|   IBIS Model for AM1802ZCE
[IBIS Ver]   3.2
[Comment Char]  |_char
[File Name]   AM1802_zce.ibs
[File Rev]   1.0
[Date]   March 8, 2013
[Source]   From Optimal Corporation's PakSi-E result.
[Notes]   Created from Freon_16x16_OSV_12172008_H_1.mcm
|   (1) AM1802 ZCE contains dual rail I/O buffers that
|   are capable of running are two different core
|   voltages depedent on the schematic hookup
|   (a) 1.8V
|   (b) 3.3V
|   (2) Specific Model Sections/Name Decoders are determined
|   based upon the value that is supplied to the
|   particular I/O buffer as well as any pull up/down
|   resistors that are selected. Refer to the Model Selecter
|   Definitions for details regarding model selection at
|   1.8V rail or the 3.3V rail.
[Disclaimer]
|   Please be aware that in the absence of a written agreement
|   Texas Instruments (TI) assumes no liability for:
|   (1) The accuracy of the IBIS models provided to your company
|   (2) The proper functioning of these Models in your design
|   or for any resulting applications;or
|   (3) Infringement of patents,copyrights, or intellectual
|   property rights resulting from your use of these models.
|   TI provides IBIS Models as a service to our customers and
|   therefore reserves the right to limit distribution of the
|   Models.
[Copyright] Copyright 2011, Texas Instruments Incorporated. All Rights Reserved
[Component]   AM1802ZCE
[Manufacturer]   Texas Instruments
[Package]
| variable   typ   min   max
R_pkg   4.15668e-001  2.28452e-002  6.49659e-001
L_pkg   3.30265e-009  8.15850e-011  6.01630e-009
C_pkg   7.30249e-013  5.00661e-013  1.13139e-012
| Note - some signal_names were truncated to meet the 80 character
|  per line limit of IBIS spec v3.2
[Pin] signal_name  model_name R_pin   L_pin   C_pin
A1   ACLKR_GP015  BC1833DV40CTPBFZ 5.91871e-001 5.89640e-009 8.85863e-013
B1   ACLKX_GP014  BC1833DV40CTPBFZ 4.86257e-001 5.42480e-009 8.43455e-013
C2   AFSR0_GP013  BC1833DV40CTPBFZ 4.95087e-001 4.50480e-009 8.94184e-013
B2   AFSX0_GP012  BC1833DV40CTPBFZ 5.24155e-001 4.89370e-009 9.02440e-013
A2   AHCLKR   BC1833DV40CTPBFZ 5.57738e-001 5.17010e-009 9.36823e-013
A3   AHCLKX   BC1833DV40CTPBFZ 6.49659e-001 6.01630e-009 1.04360e-012
D5   AMUTE   BC1833DV40CTPBFZ 5.05628e-001 3.54900e-009 1.13139e-012
F4   AMUTEIN   BC1833DV40CTPBFZ 2.70359e-001 2.09390e-009 8.60715e-013
F3   AXR00   BC1833DV40CTPBFZ 5.87268e-001 5.04320e-009 8.85130e-013
E1   AXR01   BC1833DV40CTPBFZ 5.06257e-001 4.56730e-009 7.02096e-013
D4   AXR010   BC1833DV40CTPBFZ 4.50538e-001 2.95250e-009 9.90146e-013
C5   AXR011   BC1833DV40CTPBFZ 2.58059e-001 2.51010e-009 8.40608e-013
C4   AXR012   BC1833DV40CTPBFZ 4.53251e-001 3.15490e-009 8.42999e-013
B3   AXR013   BC1833DV40CTPBFZ 4.94703e-001 4.00220e-009 7.40491e-013
B4   AXR014   BC1833DV40CTPBFZ 6.26064e-001 5.27040e-009 8.70708e-013
A4   AXR015   BC1833DV40CTPBFZ 5.69193e-001 4.65980e-009 7.60530e-013
E2   AXR02   BC1833DV40CTPBFZ 4.58046e-001 4.05840e-009 7.62216e-013
E3   AXR03   BC1833DV40CTPBFZ 6.03822e-001 5.34400e-009 9.04861e-013
D1   AXR04   BC1833DV40CTPBFZ 5.22228e-001 4.82720e-009 7.59112e-013
D3   AXR05   BC1833DV40CTPBFZ 6.17668e-001 5.68500e-009 9.46537e-013
C1   AXR06   BC1833DV40CTPBFZ 5.46060e-001 5.18360e-009 7.72304e-013
D2   AXR07   BC1833DV40CTPBFZ 4.69058e-001 4.07530e-009 8.16364e-013
E4   AXR08   BC1833DV40CTPBFZ 4.33873e-001 2.99390e-009 9.65579e-013
C3   AXR09   BC1833DV40CTPBFZ 4.41997e-001 3.42670e-009 8.54225e-013
C14  EMAA0_GP50   BC1833DV40CTPBFZ 2.98382e-001 2.12110e-009 6.59617e-013
D15  EMAA1_GP51   BC1833DV40CTPBFZ 5.42787e-001 4.38610e-009 7.97764e-013
C12  EMAA10_GP510 BC1833DV40CTPBFZ 2.66169e-001 1.88560e-009 6.21067e-013
B12  EMAA11_GP511 BC1833DV40CTPBFZ 2.63919e-001 2.25010e-009 6.03279e-013
D13  EMAA12_GP512 BC1833DV40CTPBFZ 4.96551e-001 4.38480e-009 8.15026e-013
D11  EMAA13_GP513 BC1833DV40CTPBFZ 4.28105e-001 2.84370e-009 7.34402e-013
A12  EMAA14_GP514 BC1833DV40CTPBFZ 3.52992e-001 3.00810e-009 5.84119e-013
C11  EMAA15_GP515 BC1833DV40CTPBFZ 2.52056e-001 1.79990e-009 6.53107e-013
E12  EMAA16_GP40  BC1833DV40CTPBFZ 5.25507e-001 4.62630e-009 8.90034e-013
B11  EMAA17_GP41  BC1833DV40CTPBFZ 3.48210e-001 2.51590e-009 6.11958e-013
E11  EMAA18_GP42  BC1833DV40CTPBFZ 4.54964e-001 3.32960e-009 8.69791e-013
C10  EMAA19_GP43  BC1833DV40CTPBFZ 3.76906e-001 2.39340e-009 7.09774e-013
B14  EMAA2_GP52   BC1833DV40CTPBFZ 3.90592e-001 2.72300e-009 6.24758e-013
A11  EMAA20_GP44  BC1833DV40CTPBFZ 3.45761e-001 2.96740e-009 6.10012e-013
B10  EMAA21_GP45  BC1833DV40CTPBFZ 2.46960e-001 2.00900e-009 5.42935e-013
A10  EMAA22_GP46  BC1833DV40CTPBFZ 3.33152e-001 2.60470e-009 5.37496e-013
E9   EMAA23_GP47  BC1833DV40CTPBFZ 3.19065e-001 2.29880e-009 7.32743e-013
D14  EMAA3_GP53   BC1833DV40CTPBFZ 4.79376e-001 3.69480e-009 7.71487e-013
A14  EMAA4_GP54   BC1833DV40CTPBFZ 3.97984e-001 3.13500e-009 5.42094e-013
C13  EMAA5_GP55   BC1833DV40CTPBFZ 4.22523e-001 2.74470e-009 6.79880e-013
E13  EMAA6_GP56   BC1833DV40CTPBFZ 3.48995e-001 2.90190e-009 8.13518e-013
B13  EMAA7_GP57   BC1833DV40CTPBFZ 3.66929e-001 2.60810e-009 6.24751e-013
A13  EMAA8_GP58   BC1833DV40CTPBFZ 3.72708e-001 3.04190e-009 5.38465e-013
D12  EMAA9_GP59   BC1833DV40CTPBFZ 3.33588e-001 2.40090e-009 7.00953e-013
C15  EMABA0_GP28  BC1833DV40CTPBFZ 3.18300e-001 2.38740e-009 7.10753e-013
A15  EMABA1_GP29  BC1833DV40CTPBFZ 4.17096e-001 3.30950e-009 5.86538e-013
A9   EMACASn_GP24 BC1833DV40CTPBFZ 3.54881e-001 2.82330e-009 5.65088e-013
B7   EMACLK_GP27  BC1833DV40CTPBFZ 3.56531e-001 2.34950e-009 5.60045e-013
A18  EMACS0n_GP20 BC1833DV40CTPBFZ 3.97081e-001 3.74280e-009 7.21563e-013
B17  EMACS2n_GP315 BC1833DV40CTPBFZ 5.80198e-001 5.09880e-009 8.43227e-013
A17  EMACS3n_GP314 BC1833DV40CTPBFZ 3.78016e-001 3.46170e-009 7.23538e-013
F9   EMACS4n_GP313 BC1833DV40CTPBFZ 5.19550e-001 3.90300e-009 9.18755e-013
B16  EMACS5n_GP212 BC1833DV40CTPBFZ 5.51095e-001 4.76040e-009 7.96121e-013
C9   EMAD0_GP48   BC1833DV40CTPBFZ 2.44304e-001 1.64890e-009 6.18740e-013
A8   EMAD1_GP49   BC1833DV40CTPBFZ 3.32250e-001 2.52330e-009 5.06368e-013
A7   EMAD10_GP32  BC1833DV40CTPBFZ 3.48770e-001 2.64970e-009 5.08237e-013
D6   EMAD11_GP33  BC1833DV40CTPBFZ 2.37569e-001 1.57190e-009 7.49192e-013
A6   EMAD12_GP34  BC1833DV40CTPBFZ 5.66268e-001 4.40960e-009 8.45128e-013
B6   EMAD13_GP35  BC1833DV40CTPBFZ 5.13874e-001 3.70700e-009 7.90354e-013
C7   EMAD14_GP36  BC1833DV40CTPBFZ 5.91744e-001 4.61700e-009 1.00047e-012
E6   EMAD15_GP37  BC1833DV40CTPBFZ 1.98115e-001 1.36540e-009 7.81085e-013
B8   EMAD2_GP410  BC1833DV40CTPBFZ 3.46727e-001 2.30150e-009 5.60570e-013
E8   EMAD3_GP411  BC1833DV40CTPBFZ 4.91407e-001 3.76040e-009 8.64890e-013
B5   EMAD4_GP412  BC1833DV40CTPBFZ 4.54268e-001 3.17380e-009 6.52985e-013
E7   EMAD5_GP413  BC1833DV40CTPBFZ 2.62992e-001 2.12650e-009 1.09788e-012
C6   EMAD6_GP414  BC1833DV40CTPBFZ 5.38100e-001 3.95790e-009 8.47380e-013
D7   EMAD7_GP415  BC1833DV40CTPBFZ 5.81194e-001 4.67290e-009 1.06233e-012
E10  EMAD8_GP30   BC1833DV40CTPBFZ 3.75790e-001 3.17900e-009 8.92133e-013
D9   EMAD9_GP31   BC1833DV40CTPBFZ 4.95004e-001 3.95170e-009 7.99211e-013
B15  EMAOEn_GP310 BC1833DV40CTPBFZ 2.95177e-001 2.25360e-009 5.63438e-013
A16  EMARASn_GP25 BC1833DV40CTPBFZ 4.31087e-001 3.59950e-009 5.83703e-013
D10  EMARNW_GP39  BC1833DV40CTPBFZ 4.67072e-001 3.80790e-009 7.79641e-013
D8   EMASDCKE_GP26 BC1833DV40CTPBFZ 4.66445e-001 3.42630e-009 7.54319e-013
B18  EMAWAIT0_GP38 BC1833DV40CTPBFZ 4.09634e-001 3.45430e-009 7.14985e-013
B19  EMAWAIT1_GP21 BC1833DV40CTPBFZ 4.41357e-001 4.08480e-009 8.09083e-013
B9   EMAWEn_GP311 BC1833DV40CTPBFZ 3.54014e-001 2.53790e-009 5.62877e-013
C8   EMAWEDQM0n_GP23 BC1833DV40CTPBFZ 3.74193e-001 2.37840e-009 6.26113e-013
A5   EMAWEDQM1n_GP22 BC1833DV40CTPBFZ 5.13242e-001 3.94230e-009 6.49289e-013
U7   DDRA0   BSSTL18TCSCGPBFZ 4.14960e-001 2.73750e-009 6.79471e-013
T7   DDRA1   BSSTL18TCSCGPBFZ 4.61192e-001 3.10260e-009 7.39296e-013
W6   DDRA2   BSSTL18TCSCGPBFZ 3.98765e-001 3.02010e-009 5.57871e-013
V6   DDRA3   BSSTL18TCSCGPBFZ 2.72035e-001 2.08680e-009 5.20945e-013
U5   DDRA4   BSSTL18TCSCGPBFZ 4.39992e-001 3.22490e-009 6.44839e-013
V5   DDRA5   BSSTL18TCSCGPBFZ 4.35683e-001 3.07040e-009 5.81074e-013
W5   DDRA6   BSSTL18TCSCGPBFZ 4.21472e-001 3.27020e-009 5.67079e-013
U6   DDRA7   BSSTL18TCSCGPBFZ 2.85462e-001 1.89380e-009 6.46976e-013
U4   DDRA8   BSSTL18TCSCGPBFZ 4.88010e-001 3.63800e-009 7.05605e-013
T6   DDRA9   BSSTL18TCSCGPBFZ 1.92149e-001 1.42270e-009 6.24918e-013
W4   DDRA10   BSSTL18TCSCGPBFZ 4.35328e-001 3.47630e-009 5.60660e-013
T4   DDRA11   BSSTL18TCSCGPBFZ 5.10405e-001 3.72920e-009 8.12116e-013
V4   DDRA12   BSSTL18TCSCGPBFZ 4.38115e-001 3.08480e-009 5.82197e-013
T5   DDRA13   BSSTL18TCSCGPBFZ 2.15693e-001 1.70520e-009 7.47184e-013
V8   DDRBA0   BSSTL18TCSCGPBFZ 4.80522e-001 3.52320e-009 6.92654e-013
T9   DDRBA1   BSSTL18TCSCGPBFZ 2.20318e-001 1.65540e-009 6.83534e-013
U8   DDRBA2   BSSTL18TCSCGPBFZ 4.04014e-001 2.49850e-009 6.68341e-013
U9   DDRCASn   BSSTL18TCSCGPBFZ 3.88058e-001 2.44280e-009 6.26800e-013
V7   DDRCKE   BSSTL18TCSCGPBFZ 2.57587e-001 2.00620e-009 5.46471e-013
W7   DDRCLKN   BSSTL18TCSCGPBFZ 3.64269e-001 2.70550e-009 5.00661e-013
W8   DDRCLKP   BSSTL18TCSCGPBFZ 3.53476e-001 2.69690e-009 5.06199e-013
V9   DDRCSn   BSSTL18TCSCGPBFZ 3.47483e-001 2.33680e-009 5.61910e-013
U15  DDRD0   BSSTL18TCSCGPBFZ 5.03067e-001 4.08480e-009 6.88721e-013
U14  DDRD1   BSSTL18TCSCGPBFZ 4.44055e-001 3.34930e-009 6.99179e-013
V14  DDRD2   BSSTL18TCSCGPBFZ 4.43485e-001 3.67420e-009 6.49287e-013
U13  DDRD3   BSSTL18TCSCGPBFZ 4.23858e-001 3.01220e-009 6.42646e-013
V13  DDRD4   BSSTL18TCSCGPBFZ 2.95715e-001 2.54430e-009 6.14396e-013
V12  DDRD5   BSSTL18TCSCGPBFZ 3.88855e-001 2.74710e-009 5.41742e-013
W12  DDRD6   BSSTL18TCSCGPBFZ 3.67182e-001 2.92840e-009 5.28344e-013
W11  DDRD7   BSSTL18TCSCGPBFZ 2.56622e-001 2.82530e-009 6.12911e-013
T13  DDRD8   BSSTL18TCSCGPBFZ 4.76155e-001 3.51100e-009 8.24674e-013
T11  DDRD9   BSSTL18TCSCGPBFZ 4.46810e-001 3.14220e-009 7.61080e-013
T10  DDRD10   BSSTL18TCSCGPBFZ 3.12174e-001 2.45150e-009 6.81267e-013
T12  DDRD11   BSSTL18TCSCGPBFZ 4.66794e-001 3.38780e-009 8.50234e-013
U10  DDRD12   BSSTL18TCSCGPBFZ 3.86652e-001 2.58760e-009 6.64029e-013
V10  DDRD13   BSSTL18TCSCGPBFZ 3.78944e-001 2.51470e-009 6.06810e-013
U11  DDRD14   BSSTL18TCSCGPBFZ 4.74936e-001 3.29650e-009 8.05328e-013
W10  DDRD15   BSSTL18TCSCGPBFZ 3.79744e-001 3.73260e-009 6.60169e-013
W13  DDRDQM0n   BSSTL18TCSCGPBFZ 3.94835e-001 3.04360e-009 5.62703e-013
R10  DDRDQM1n   BSSTL18TCSCGPBFZ 4.61673e-001 3.54330e-009 8.26589e-013
W9   DDRRASn   BSSTL18TCSCGPBFZ 3.50051e-001 2.72800e-009 5.47279e-013
R11  DDRDQGATE0   BSSTL18TCSCGPBFZ 4.90814e-001 3.50590e-009 8.76801e-013
R12  DDRDQGATE1   BSSTL18TCSCGPBFZ 5.15291e-001 3.70680e-009 9.84983e-013
T8   DDRWEn   BSSTL18TCSCGPBFZ 4.42497e-001 2.97360e-009 6.63102e-013
T14  DDRDQS0   BSSTL18TCSCGPBFZ 4.80092e-001 3.48030e-009 7.80760e-013
V11  DDRDQS1   BSSTL18TCSCGPBFZ 4.22650e-001 3.29520e-009 6.81403e-013
J16  EMU0   BC1833DV40CTPBFZ 2.54325e-001 1.81840e-009 7.85509e-013
K16  EMU1   BC1833DV40CTPBFZ 4.29846e-001 3.27960e-009 8.14633e-013
K4   GP61   BC1833DV40CTPBFZ 3.63614e-001 2.49020e-009 8.31825e-013
J3   GP62   BC1833DV40CTPBFZ 2.73739e-001 2.52640e-009 7.69287e-013
K3   GP63   BC1833DV40CTPBFZ 3.69454e-001 2.75510e-009 7.14832e-013
H3   GP64   BC1833DV40CTPBFZ 5.80089e-001 5.21570e-009 8.91399e-013
F2   GP810   BC1833DV40CTPBFZ 4.49068e-001 3.95750e-009 7.41073e-013
F1   GP811   BC1833DV40CTPBFZ 4.97064e-001 4.59930e-009 7.63107e-013
G3   GP812   BC1833DV40CTPBFZ 4.22225e-001 3.12280e-009 9.06650e-013
J4   GP813   BC1833DV40CTPBFZ 4.18358e-001 2.77620e-009 8.64397e-013
G2   GP814   BC1833DV40CTPBFZ 4.46474e-001 3.75040e-009 7.54261e-013
G1   GP815   BC1833DV40CTPBFZ 4.80067e-001 4.12220e-009 6.81038e-013
G4   GP88   BC1833DV40CTPBFZ 3.97460e-001 2.83360e-009 8.04305e-013
H4   GP89   BC1833DV40CTPBFZ 4.23690e-001 2.97660e-009 8.22397e-013
R5   GP60   BC1833DV40CTPBFZ 2.45883e-001 2.09100e-009 8.01025e-013
W1   GP78   BC1833DV40CTPBFZ 4.78964e-001 4.27560e-009 6.54315e-013
W2   GP79   BC1833DV40CTPBFZ 4.54813e-001 3.82070e-009 6.79498e-013
T2   GP72   BC1833DV40CTPBFZ 4.36957e-001 3.45270e-009 5.91877e-013
T3   GP73   BC1833DV40CTPBFZ 4.16931e-001 3.05630e-009 6.29650e-013
R1   GP74   BC1833DV40CTPBFZ 4.54506e-001 3.65190e-009 6.34173e-013
R2   GP75   BC1833DV40CTPBFZ 4.20647e-001 3.27220e-009 7.29881e-013
R3   GP76   BC1833DV40CTPBFZ 3.26617e-001 2.78190e-009 6.90042e-013
P4   GP77   BC1833DV40CTPBFZ 4.14093e-001 2.81750e-009 7.64469e-013
W3   GP710   BC1833DV40CTPBFZ 2.28452e-002 1.01420e-010 5.62555e-013
V1   GP711   BC1833DV40CTPBFZ 4.77687e-001 4.00580e-009 6.74578e-013
V2   GP712   BC1833DV40CTPBFZ 4.48597e-001 3.75400e-009 6.51164e-013
V3   GP713   BC1833DV40CTPBFZ 4.36018e-001 3.43390e-009 7.00041e-013
U1   GP714   BC1833DV40CTPBFZ 4.80254e-001 3.78490e-009 6.52073e-013
U2   GP715   BC1833DV40CTPBFZ 4.40999e-001 3.40200e-009 6.15258e-013
U3   GP70   BC1833DV40CTPBFZ 4.34081e-001 3.33150e-009 6.89105e-013
T1   GP71   BC1833DV40CTPBFZ 4.87422e-001 3.88830e-009 5.92797e-013
J17  NMIn   IC1833DVTPBFZP18LL 3.65961e-001 2.64340e-009 6.81345e-013
K14  RESETn   IHHV1833DVTP18 3.13948e-001 1.92720e-009 9.39463e-013
K17  GP80   BC1833DV40CTPBFZ 4.98560e-001 4.09850e-009 7.97021e-013
D19  EPWM0A   BC1833DV40CTPBFZ 5.47450e-001 4.73470e-009 7.69394e-013
C17  EPWM0B   BC1833DV40CTPBFZ 2.77268e-001 2.63370e-009 7.30178e-013
D17  GP16   BC1833DV40CTPBFZ 4.00877e-001 2.84850e-009 6.63256e-013
E16  GP17   BC1833DV40CTPBFZ 1.85753e-001 1.58290e-009 7.38386e-013
D16  GP81   BC1833DV40CTPBFZ 2.94303e-001 2.04320e-009 6.93329e-013
E17  GP82   BC1833DV40CTPBFZ 4.47987e-001 3.34480e-009 7.84496e-013
D18  GP83   BC1833DV40CTPBFZ 4.37452e-001 3.53960e-009 6.89681e-013
C19  GP84   BC1833DV40CTPBFZ 4.72581e-001 3.82440e-009 6.65189e-013
C18  GP85   BC1833DV40CTPBFZ 4.70155e-001 3.77380e-009 6.89104e-013
C16  GP86   BC1833DV40CTPBFZ 2.76089e-001 2.46530e-009 7.57539e-013
G19  SPI1CLK_GP213 BC1833DV40CTPBFZ 4.69262e-001 4.17240e-009 7.11445e-013
H16  SPI1ENAn_GP212 BC1833DV40CTPBFZ 2.65537e-001 2.13550e-009 7.16472e-013
E19  SPI1SCS0n   BC1833DV40CTPBFZ 4.90496e-001 4.15100e-009 7.37763e-013
F18  SPI1SCS1n   BC1833DV40CTPBFZ 4.59876e-001 3.78990e-009 7.28257e-013
F19  SPI1SCS2n   BC1833DV40CTPBFZ 4.93949e-001 4.19790e-009 7.59046e-013
E18  SPI1SCS3n   BC1833DV40CTPBFZ 3.81442e-001 3.01750e-009 6.17218e-013
F16  SPI1SCS4n   BC1833DV40CTPBFZ 3.91821e-001 2.59160e-009 7.64737e-013
F17  SPI1SCS5n   BC1833DV40CTPBFZ 3.81978e-001 2.67900e-009 6.57715e-013
G18  SPI1SCS6n   BC1833DV40CTPBFZ 4.07238e-001 3.79210e-009 7.95139e-013
G16  SPI1SCS7n   BC1833DV40CTPBFZ 2.69265e-001 1.90170e-009 7.00785e-013
G17  SPI1SIMO_GP210 BC1833DV40CTPBFZ 3.72117e-001 2.60560e-009 6.80138e-013
H17  SPI1SOMI_GP211 BC1833DV40CTPBFZ 4.56903e-001 3.42860e-009 7.28034e-013
J15  TCK   IC1833DVTPBFZP18LL 2.57521e-001 1.72010e-009 7.51806e-013
M16  TDI   IC1833DVTPBFZP18LL 5.58912e-001 5.27220e-009 1.06666e-012
J18  TDO   BC1833DV40CTPBFZ 3.51274e-001 2.87560e-009 6.76444e-013
L16  TMS   IC1833DVTPBFZP18LL 3.99407e-001 2.92060e-009 8.37004e-013
L17  TRSTn   IC1833DVTPBFZP18LL 3.86978e-001 3.09900e-009 7.62159e-013
T17  UHPIHASn   BC1833DV40CTPBFZ 3.86492e-001 2.71460e-009 7.41946e-013
U17  UHPIHCNTL0   BC1833DV40CTPBFZ 2.42945e-002 8.15850e-011 8.17122e-013
W15  UHPIHCNTL1   BC1833DV40CTPBFZ 4.27573e-001 3.54430e-009 5.42549e-013
W14  UHPIHCSn   BC1833DV40CTPBFZ 3.48379e-001 3.02510e-009 5.61183e-013
P17  UHPIHD0   BC1833DV40CTPBFZ 5.04430e-001 4.02180e-009 9.65050e-013
R15  UHPIHD1   BC1833DV40CTPBFZ 4.61967e-001 3.22070e-009 9.22461e-013
W17  UHPIHD10   BC1833DV40CTPBFZ 5.06372e-001 4.43790e-009 6.29295e-013
V17  UHPIHD11   BC1833DV40CTPBFZ 5.14141e-001 4.40180e-009 6.46147e-013
W16  UHPIHD12   BC1833DV40CTPBFZ 4.47674e-001 3.61480e-009 5.80945e-013
R14  UHPIHD13   BC1833DV40CTPBFZ 2.29936e-001 1.93580e-009 9.83864e-013
V16  UHPIHD14   BC1833DV40CTPBFZ 4.88188e-001 3.91970e-009 6.17589e-013
U18  UHPIHD15   BC1833DV40CTPBFZ 5.62311e-001 4.83050e-009 8.64648e-013
R19  UHPIHD2   BC1833DV40CTPBFZ 5.16823e-001 4.57930e-009 7.51770e-013
R18  UHPIHD3   BC1833DV40CTPBFZ 5.00110e-001 4.15440e-009 7.75793e-013
T16  UHPIHD4   BC1833DV40CTPBFZ 2.66853e-001 2.25470e-009 8.85923e-013
U19  UHPIHD5   BC1833DV40CTPBFZ 5.90890e-001 5.06810e-009 8.95998e-013
V19  UHPIHD6   BC1833DV40CTPBFZ 5.79160e-001 4.93500e-009 7.59523e-013
V18  UHPIHD7   BC1833DV40CTPBFZ 5.37053e-001 4.49240e-009 8.46758e-013
W19  UHPIHD8   BC1833DV40CTPBFZ 5.52593e-001 5.15440e-009 7.41144e-013
W18  UHPIHD9   BC1833DV40CTPBFZ 5.25636e-001 4.65020e-009 7.16361e-013
V15  UHPIHDS1n   BC1833DV40CTPBFZ 3.19300e-001 2.53200e-009 7.20635e-013
T18  UHPIHDS2n   BC1833DV40CTPBFZ 3.90741e-001 3.11240e-009 6.27607e-013
U16  UHPIHHWIL   BC1833DV40CTPBFZ 5.17218e-001 4.36310e-009 7.63222e-013
R16  UHPIHINTn   BC1833DV40CTPBFZ 4.10882e-001 2.49400e-009 7.51548e-013
R17  UHPIHRDYn   BC1833DV40CTPBFZ 3.95791e-001 2.69860e-009 8.08520e-013
T15  UHPIHRWn   BC1833DV40CTPBFZ 3.77610e-001 2.93410e-009 7.45095e-013
K18  USB0DRVVBUS  BC1833DV40CTPBFZ 3.81954e-001 3.14290e-009 6.88529e-013
[Model Selector] IHHV1833DVTP18
|  This seciton is used to determine the IBIS model to use depending
|  on which voltage is supplied to the Dual Voltage I/O Buffers
HV1833DVTP18_7LM_1P8   Dual Voltage I/O Buffer with 1.8V External Supply
HV1833DVTP18_7LM_3P3   Dual Voltage I/O Buffer with 3.3V External Supply
[Model Selector] IC1833DVTPBFZP18LL
|  This seciton is used to determine which IBIS Model is to be used
|  for the pins depending on the functionality required by the user's
|  application.
BFZP18LL_!PI_LOW_1P8  Cell operated at 1.8(nom)
|IC1833DVTPBFZP18LL_!PI_LOW_1P8;
|BUFFER WITH WEAK_PULLDOWN_ON NOMINAL CURRENT OF 100UA WHEN PAD=VDDS
FZP18LL_!PI_HIGH_1P8  Cell operated at 1.8(nom)
|IC1833DVTPBFZP18LL_!PI_HIGH_1P8;
|BUFFER WITH WEAK_PULLUP_ON NOMINAL CURRENT OF 100UA WHEN PAD=0
3DVTPBFZP18LL_PI_1P8  Cell operated at 1.8(nom)
|IC1833DVTPBFZP18LL_PI_1P8;
|BUFFER IN NORMAL MODE WITH PULLUP AND PULLDOWN OFF
BFZP18LL_!PI_LOW_3P3  Cell operated at 3.3(nom)
|IC1833DVTPBFZP18LL_!PI_LOW_3P3;
|BUFFER WITH WEAK_PULLDOWN_ON NOMINAL CURRENT OF 100UA WHEN PAD=VDDS
FZP18LL_!PI_HIGH_3P3  Cell operated at 3.3(nom)
|IC1833DVTPBFZP18LL_!PI_HIGH_3P3;
|BUFFER WITH WEAK_PULLUP_ON NOMINAL CURRENT OF 100UA WHEN PAD=0
3DVTPBFZP18LL_PI_3P3  Cell operated at 3.3(nom)
|IC1833DVTPBFZP18LL_PI_3P3;
|BUFFER IN NORMAL MODE WITH PULLUP AND PULLDOWN OFF
[Model Selector] BC1833DV40CTPBFZ
|  This seciton is used to determine the IBIS model to use depending
|  on which voltage is supplied to the Dual Voltage I/O Buffers
18LL_X50_!PI_LOW_1P8  Cell operated at 1.8(nom)
|BC1833DV40CTPBFZ_!PI_LOW_1P8;
|BUFFER WITH WEAK_PULLDOWN_ON NOMINAL CURRENT OF 100UA WHEN PAD=VDDS
8LL_X50_!PI_HIGH_1P8  Cell operated at 1.8(nom)
|BC1833DV40CTPBFZ_!PI_HIGH_1P8;
|BUFFER WITH WEAK_PULLUP_ON NOMINAL CURRENT OF 100UA WHEN PAD=0
PBFZP18LL_X50_PI_1P8  Cell operated at 1.8(nom)
|BC1833DV40CTPBFZ_PI_1P8;
|BUFFER IN NORMAL MODE WITH PULLUP AND PULLDOWN OFF
18LL_X50_!PI_LOW_3P3  Cell operated at 3.3(nom)
|BC1833DV40CTPBFZ_!PI_LOW_3P3;
|BUFFER WITH WEAK_PULLDOWN_ON NOMINAL CURRENT OF 100UA WHEN PAD=VDDS
8LL_X50_!PI_HIGH_3P3  Cell operated at 3.3(nom)
|BC1833DV40CTPBFZ_!PI_HIGH_3P3;
|BUFFER WITH WEAK_PULLUP_ON NOMINAL CURRENT OF 100UA WHEN PAD=0
PBFZP18LL_X50_PI_3P3  Cell operated at 3.3(nom)
|BC1833DV40CTPBFZ_PI_3P3;
|BUFFER IN NORMAL MODE WITH PULLUP AND PULLDOWN OFF
[Model Selector] BSSTL18TCSCGPBFZ
NOSR0_NOTERM_1P8  Cell operated at 1.8(nom)
|NOSR0_NOTERM_1P8
|BUFFER OPERATING AT FAST MODE WITH 1.8V SUPPLY WITH +/-10% VARIATION
NOSR0_NOTERM_0.1_1P8  Cell operated at 1.8(nom)
| Models and submodels in the file (16): HV1833DVTP18_7LM_1P8 (Input), HV1833DVTP18_7LM_3P3 (Input), BFZP18LL_!PI_LOW_1P8 (Input), FZP18LL_!PI_HIGH_1P8 (Input), 3DVTPBFZP18LL_PI_1P8 (Input), BFZP18LL_!PI_LOW_3P3 (Input), FZP18LL_!PI_HIGH_3P3 (Input), 3DVTPBFZP18LL_PI_3P3 (Input), NOSR0_NOTERM_1P8 (3-state), NOSR0_NOTERM_0.1_1P8 (3-state), 18LL_X50_!PI_LOW_1P8 (I/O), 8LL_X50_!PI_HIGH_1P8 (I/O), PBFZP18LL_X50_PI_1P8 (I/O), 18LL_X50_!PI_LOW_3P3 (I/O), 8LL_X50_!PI_HIGH_3P3 (I/O), PBFZP18LL_X50_PI_3P3 (I/O)
